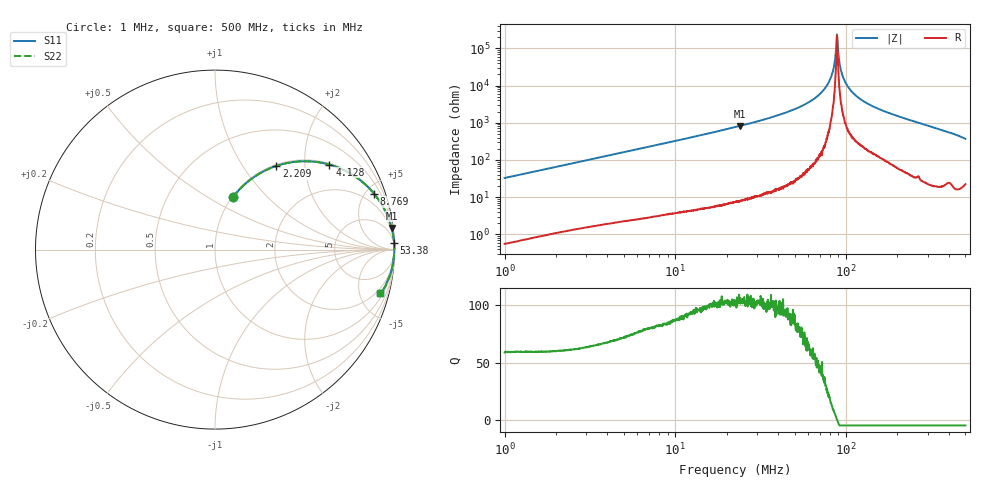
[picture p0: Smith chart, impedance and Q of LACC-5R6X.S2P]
!s-Parameter Generated by FASTRON Sdn. Bhd.
!FASTRON P/N : LACC-5R6X
!Keysight Technologies,E4991B,MY54100416,A.01.15
!Date: Wed Mar 18 09:16:53 2026
!Version  : Rev00 Wed Mar 18 09:16:53 2026
!Data & Calibration Information:
!PortZ  Port1:50+j0  Port2:50+j0
!When reading, reference impedance value at option line is always used.
!Remarks : This data is being provided solely for informational purposes.
!Freq	S11	S21	S12	S22
# Hz S dB R 50
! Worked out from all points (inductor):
!   1601 points, 1 MHz to 500 MHz, reference 50 ohm
!   read as one part in series: L = 5.19 uH near 1.032 MHz
!   highest Q = 106 at 23.79 MHz (marker M1), where L = 5.46 uH
!   self-resonance near 88.44 MHz
!   S11 on the Smith chart (normalised r, x): 1 MHz: 1.01, +0.65; 2.209 MHz: 1.02, +1.43; 4.128 MHz: 1.04, +2.66; 8.769 MHz: 1.07, +5.67; 53.38 MHz: 2, +53; 500 MHz: 1.45, -7.38
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1000000  -10.19 71.0  -0.48 -18.0  -0.48 -18.0  -10.19 71.0
2208608  -4.76 53.7  -1.87 -35.3  -1.87 -35.3  -4.76 53.7
2820919  -3.49 47.1  -2.70 -42.0  -2.70 -42.0  -3.49 47.1
4127647  -2.00 36.6  -4.49 -52.6  -4.49 -52.6  -2.00 36.6
7957584  -0.65 21.2  -8.85 -68.1  -8.85 -68.1  -0.65 21.2
8769052  -0.54 19.4  -9.59 -70.0  -9.59 -70.0  -0.54 19.4
2.236068e7  -0.09 7.5  -17.70 -81.9  -17.70 -81.9  -0.09 7.5
2.37944e7  -0.07 7.0  -18.30 -82.5  -18.30 -82.5  -0.07 7.0
5.337536e7  -0.01 2.2  -28.43 -87.1  -28.43 -87.1  -0.01 2.2
6.307767e7  -0.01 1.4  -32.08 -87.6  -32.08 -87.6  -0.01 1.4
7.226293e7  -0.00 0.9  -36.56 -88.0  -36.56 -88.0  -0.00 0.9
7.901568e7  -0.00 0.5  -41.57 -87.0  -41.57 -87.0  -0.00 0.5
8.310792e7  -0.00 0.3  -46.63 -84.7  -46.63 -84.7  -0.00 0.3
8.673569e7  -0.00 0.1  -56.11 -75.4  -56.11 -75.4  -0.00 0.1
8.878078e7  -0.00 -0.0  -65.88 15.3  -65.88 15.3  -0.00 -0.0
9.052181e7  -0.00 -0.1  -55.60 74.2  -55.60 74.2  -0.00 -0.1
9.301677e7  -0.00 -0.2  -48.78 81.9  -48.78 81.9  -0.00 -0.2
9.595246e7  -0.00 -0.3  -44.60 84.3  -44.60 84.3  -0.00 -0.3
1.065617e8  -0.01 -0.8  -37.33 85.6  -37.33 85.6  -0.01 -0.8
1.299065e8  -0.02 -1.6  -30.94 85.2  -30.94 85.2  -0.02 -1.6
1.77937e8  -0.03 -3.1  -25.30 84.2  -25.30 84.2  -0.03 -3.1
5e8  -0.44 -14.9  -11.79 71.7  -11.79 71.7  -0.44 -14.9
